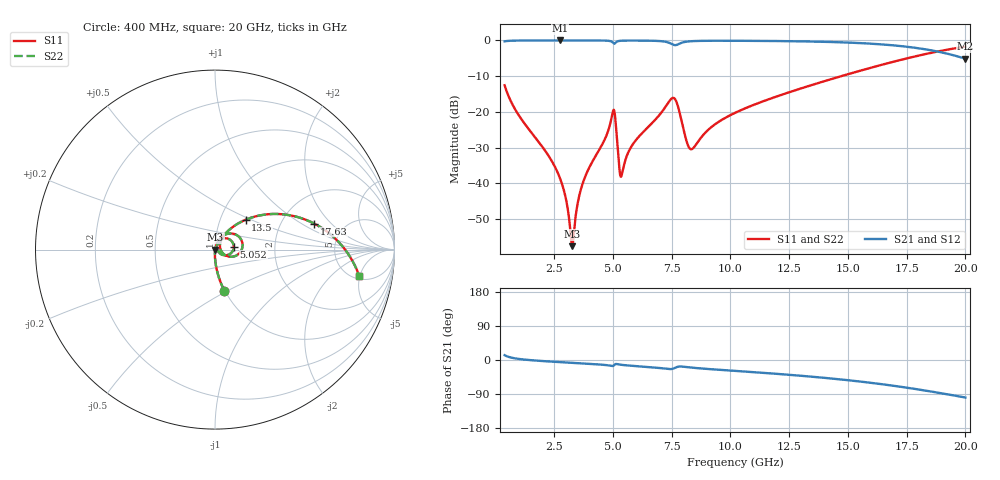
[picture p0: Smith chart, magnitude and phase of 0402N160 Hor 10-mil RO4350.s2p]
# GHz S MA R 50
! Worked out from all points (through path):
!   1960 points, 400 MHz to 20 GHz, reference 50 ohm
!   highest |S21| = -0.01 dB at 2.751 GHz (marker M1); lowest = -5.1 dB at 20 GHz (marker M2)
!   group delay of S21, straight-line fit = 13 ps
!   lowest |S11| = -57.6 dB at 3.271 GHz (marker M3), VSWR 1.00, Z = 50.1 - j0.0279 ohm
!   |S11| at or under -10 dB: start of sweep to 14.72 GHz
!   |S22| runs from -57.6 to -1.7 dB; largest |S21 - S12| = 0
!   S11 on the Smith chart (normalised r, x): 400 MHz: 0.99, -0.48; 5.052 GHz: 1.23, +0.04; 13.5 GHz: 1.32, +0.47; 17.63 GHz: 3.06, +1.31; 20 GHz: 5.47, -4.92
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0.4  0.2352 -77.2  0.9713 12.7  0.9713 12.7  0.2352 -77.2
1.100357  0.08012 -87.3  0.9959 2.1  0.9959 2.1  0.08012 -87.3
2.7512  0.01186 -90.0  0.9986 -5.6  0.9986 -5.6  0.01186 -90.0
3.001327  0.006183 -85.1  0.9986 -6.5  0.9986 -6.5  0.006183 -85.1
3.271465  0.001315 -12.2  0.9985 -7.5  0.9985 -7.5  0.001315 -12.2
3.671669  0.008813 71.4  0.9983 -8.9  0.9983 -8.9  0.008813 71.4
5.052374  0.1062 9.3  0.9014 -14.0  0.9014 -14.0  0.1062 9.3
5.122409  0.07167 -26.1  0.9305 -10.6  0.9305 -10.6  0.07167 -26.1
5.282491  0.01585 -19.4  0.9841 -12.0  0.9841 -12.0  0.01585 -19.4
5.372537  0.01274 27.6  0.99 -12.8  0.99 -12.8  0.01274 27.6
5.832772  0.03432 67.5  0.9948 -15.3  0.9948 -15.3  0.03432 67.5
6.943338  0.08704 59.9  0.9818 -20.8  0.9818 -20.8  0.08704 59.9
7.623686  0.1541 6.3  0.8607 -21.5  0.8607 -21.5  0.1541 6.3
8.163961  0.03652 -14.0  0.9633 -18.8  0.9633 -18.8  0.03652 -14.0
8.344053  0.02991 15.2  0.9751 -20.0  0.9751 -20.0  0.02991 15.2
9.184482  0.06074 56.8  0.9884 -24.3  0.9884 -24.3  0.06074 56.8
10.205  0.09686 57.5  0.9884 -28.7  0.9884 -28.7  0.09686 57.5
13.46667  0.2373 44.4  0.9644 -44.0  0.9644 -44.0  0.2373 44.4
13.49668  0.239 44.2  0.9639 -44.2  0.9639 -44.2  0.239 44.2
16.73834  0.4834 22.5  0.8641 -66.2  0.8641 -66.2  0.4834 22.5
17.62879  0.5726 14.6  0.8065 -74.2  0.8065 -74.2  0.5726 14.6
20  0.8179 -10.5  0.5534 -99.0  0.5534 -99.0  0.8179 -10.5
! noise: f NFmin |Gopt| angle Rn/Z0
0.4  0.001308  0.7927  1.294  0.001302
2.571  0.004465  0.6427  5.989  0.002357
4.752  0.01537  0.7914  10.8  0.01506
6.933  0.02533  0.814  15.72  0.02792
9.104  0.02453  0.7574  20.57  0.01982
11.29  0.02108  0.6704  24.9  0.01175
13.47  0.02454  0.6668  29.14  0.01327
15.64  0.03124  0.6954  33.37  0.01842
17.82  0.04327  0.7467  37.74  0.03084
20  0.06895  0.8186  42.38  0.06929
